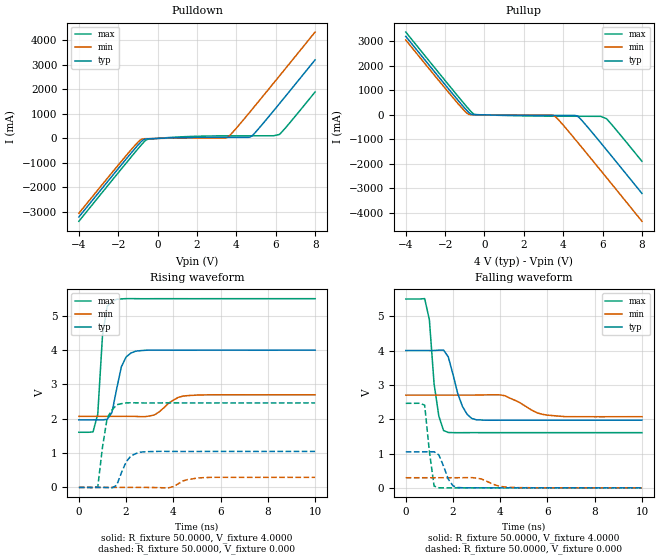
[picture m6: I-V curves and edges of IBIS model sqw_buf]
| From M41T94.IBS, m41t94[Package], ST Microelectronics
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|   Model sqw_buf
[Model]   sqw_buf
Model_type   Output
Polarity   Non-Inverting
Vmeas =   1.5000V
Cref =1.000e-10F
Rref =   0.6450k
Vref =   1.7300V
C_comp   5.1600pF   4.9600pF   5.3500pF
[Temperature Range]   27.0000   85.0000   -40.0000
[Voltage Range]   4.0000V   2.7000V   5.5000V
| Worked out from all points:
|   slope of the pulldown table from 0 to 0.6 V, typ, clamps not added: 31.7 ohm
|   slope of the pullup table from 0 to 0.6 V, typ, clamps not added: 80.2 ohm
|   rising waveform, R_fixture 50.0000, V_fixture 4.0000: 20-80 % time 398ps typ, 690ps min, 247ps max; typ from 1.97 V to 4 V
|   rising waveform, R_fixture 50.0000, V_fixture 0.000: 20-80 % time 431ps typ, 583ps min, 304ps max; typ from 0 V to 1.05 V
|   falling waveform, R_fixture 50.0000, V_fixture 4.0000: 20-80 % time 511ps typ, 991ps min, 318ps max; typ from 4 V to 1.97 V
|   falling waveform, R_fixture 50.0000, V_fixture 0.000: 20-80 % time 370ps typ, 637ps min, 247ps max; typ from 1.05 V to 0 V
[Pulldown]
| voltage   I(typ)   I(min)   I(max)
-4V       -3.208A    -3.056A    -3.384A
-1.3V     -554.5mA   -418.8mA   -715.9mA
-900mV    -185.5mA   -76.85mA   -332.7mA
-600mV    -22.02mA   -10.78mA   -74.18mA
1V        28.1mA     10.99mA    56.17mA
3.4V      43.8mA     13.72mA    104.5mA
3.6V      43.96mA    76.02mA    105.1mA
4.7V      55.39mA    1.088A     107.3mA
5V        275.8mA    1.381A     107.7mA
5.9V      1.135A     2.265A     109mA
6.2V      1.429A     2.561A     165.8mA
8V        3.208A     4.345A     1.896A
[Pullup]
| voltage   I(typ)   I(min)   I(max)
-4V       3.207A     3.056A     3.383A
-1V       272.5mA    150.4mA    425.9mA
-800mV    100.2mA    20.4mA     238.1mA
-700mV    33.98mA    5.777mA    148.5mA
-500mV    7.158mA    3.443mA    17.28mA
3.5V      -21.67mA   -21.33mA   -51.98mA
3.8V      -21.97mA   -236.2mA   -53.31mA
4.7V      -41.43mA   -1.088A    -56.35mA
5V        -273.8mA   -1.381A    -57.06mA
5.9V      -1.135A    -2.266A    -58.75mA
6.2V      -1.429A    -2.562A    -155.2mA
8V        -3.208A    -4.345A    -1.896A
[Ramp]
| variable   typ   min   max
dV/dt_r   2.1420/0.8261n   1.2349/2.2003n   3.1094/0.4008n
dV/dt_f   2.2998/0.4649n   1.4757/1.1708n   3.2278/0.2272n
R_load = 0.6450k
[Rising Waveform]
R_fixture = 50.0000
V_fixture = 4.0000
V_fixture_min = 2.7000
V_fixture_max = 5.5000
| time   V(typ)   V(min)   V(max)
0s        1.97V      2.072V     1.607V
600ps     1.97V      2.072V     1.619V
800ps     1.97V      2.072V     2.14V
1ns       1.967V     2.072V     4.432V
1.2ns     1.986V     2.072V     5.278V
1.4ns     2.182V     2.072V     5.409V
1.8ns     3.518V     2.072V     5.494V
2.4ns     3.97V      2.069V     5.501V
4.4ns     3.999V     2.66V      5.5V
10ns      4V         2.7V       5.5V
[Rising Waveform]
R_fixture = 50.0000
V_fixture = 0.000
V_fixture_min = 0.000
V_fixture_max = 0.000
| time   V(typ)   V(min)   V(max)
0s        1.561nV    1.573nV    1.394nV
800ps     -12.37uV   1.934uV    17.87mV
1ns       180.8uV    1.554uV    1.176V
1.2ns     -2.744mV   100.8nV    2.03V
1.6ns     62.7mV     -4.481uV   2.41V
2ns       743.2mV    -5.712uV   2.463V
2.6ns     1.028V     278.7uV    2.462V
3.8ns     1.05V      -10.4mV    2.463V
5.2ns     1.048V     282mV      2.462V
10ns      1.049V     293.9mV    2.463V
[Falling Waveform]
R_fixture = 50.0000
V_fixture = 4.0000
V_fixture_min = 2.7000
V_fixture_max = 5.5000
| time   V(typ)   V(min)   V(max)
0s        4V         2.7V       5.5V
800ps     4V         2.7V       5.512V
1ns       4V         2.7V       4.896V
1.2ns     4.001V     2.7V       3.026V
1.4ns     4.01V      2.7V       2.091V
1.6ns     4.012V     2.7V       1.669V
2.4ns     2.371V     2.7V       1.607V
2.8ns     2.019V     2.7V       1.608V
6ns       1.97V      2.117V     1.607V
10ns      1.97V      2.072V     1.607V
[Falling Waveform]
R_fixture = 50.0000
V_fixture = 0.000
V_fixture_min = 0.000
V_fixture_max = 0.000
| time   V(typ)   V(min)   V(max)
0s        1.048V     293.9mV    2.462V
800ps     1.049V     294mV      2.41V
1ns       1.05V      294.1mV    1.059V
1.2ns     1.05V      294.2mV    51.27mV
1.4ns     960.4mV    294.3mV    1.689mV
1.8ns     253.1mV    294.3mV    -115.7uV
2.2ns     10.18mV    294.3mV    18.99uV
3ns       26.24uV    283.7mV    -48.64uV
4.4ns     -17.54uV   13.59mV    54.44uV
10ns      46.82uV    -5.63uV    31.51uV
